(* Logix 5000 AddOnInstructionDefinition export Banner_IOLM_Param_A2_v4; software revision 36.00 *)

TYPE Banner_IOL_Port_v4 :   // UDT that has all of the data items necessary to communicate with a specific Port on a IO-Link Master
STRUCT
   Port_Controlled : INT;   // Each bit represents a port on an IO-Link Master. Set to 1 to tell AOI to control that port.
   Port_Activate : INT;   // Each bit represents a port on an IO-Link Master. When ON that port will process any commands in queue.
   Port_Read : INT;   // Each bit represents a port on an IO-Link Master. Used to determine when device AOI has requested a Read command.
   Port_Write : INT;   // Each bit represents a port on an IO-Link Master. Used to determine when device AOI has requested a Write command.
   Port_RW_Complete : INT;   // Each bit represents a port on an IO-Link Master. Tells device AOI that Read or Write request has been completed.
   Port_Device_Read : INT;
   Data_Transfer : SINT[190];   // Array to transfer data from IO-Master to device AOIs.
END_STRUCT
END_TYPE

TYPE Banner_IOLM_EL_v4 :   // Error Log for Messages to IOLM.
STRUCT
   RW : SINT;   // 0 = Read, 1 = Write.
   Port : SINT;   // Port number that generated error.
   Index : INT;   // IO-Link Index for generated error.
END_STRUCT
END_TYPE

TYPE Banner_IOLM_v4 :   // UDT to control IO-Link Masters.
STRUCT
   Message_Source_Data : SINT[190];
   Message_Destination_Data : SINT[190];
   Error_Log : Banner_IOLM_EL_v4[10];
   Error_Write_Retry : BOOL;
   Num_Error_MSGS : DINT;
   IO_Link_Master_Busy : BOOL;   // 0 = While waiting for a command, 1 = Processing command
   AOI_Reset : BOOL;
   Port_Data : Banner_IOL_Port_v4;   // All of the necessary data to work with the various ports of the IO-Link Master.
   Halt_Operation : BOOL;   // When parameter is 1 the AOI is halted as next available time frame.
   AOI_Halted : BOOL;   // AOI is in standby mode until Halt Operation tag is set back to 0.
END_STRUCT
END_TYPE

ADD_ON_INSTRUCTION Banner_IOLM_Param_A2_v4   (* revision 4.1, vendor Banner Engineering *)
// AOI that controls an Allen Bradley IO-Link Master with Banner devices for parameter data operations. Created for use with the 5032-8IOLM units only.
VAR_IN_OUT
   Message_Read : MESSAGE; {required}   // Message used to gather data from a device plugged into an Allen Bradley IO-Link Master.
   Message_Write : MESSAGE; {required}   // Message used to send parameter updates to a device plugged into an Allen Bradley IO-Link Master.
   IOLM : Banner_IOLM_v4; {required}
   ISDU_Path : STRING[8]; {required}
END_VAR
VAR_OUTPUT
   Done : BOOL; {visible}
   Busy : BOOL; {visible}
   Error : BOOL; {visible}
END_VAR
VAR
   Lock : DINT; {access None}
   Byte_Length : SINT; {access None}
   Current_Port : INT; {access None}   // Current port to communicate with via the IO-Link Master.
   Array_Index : DINT; {access None}
   Data_Index : DINT; {access None}
   Message_Timer : TIMER := (PRE := 100); {access None}
   Error_Index : DINT; {access None}
   Message_Timer2 : TIMER := (PRE := 5000); {access None}
   Temp_Index : INT; {access None}
END_VAR

ROUTINE Logic   (* ladder *)
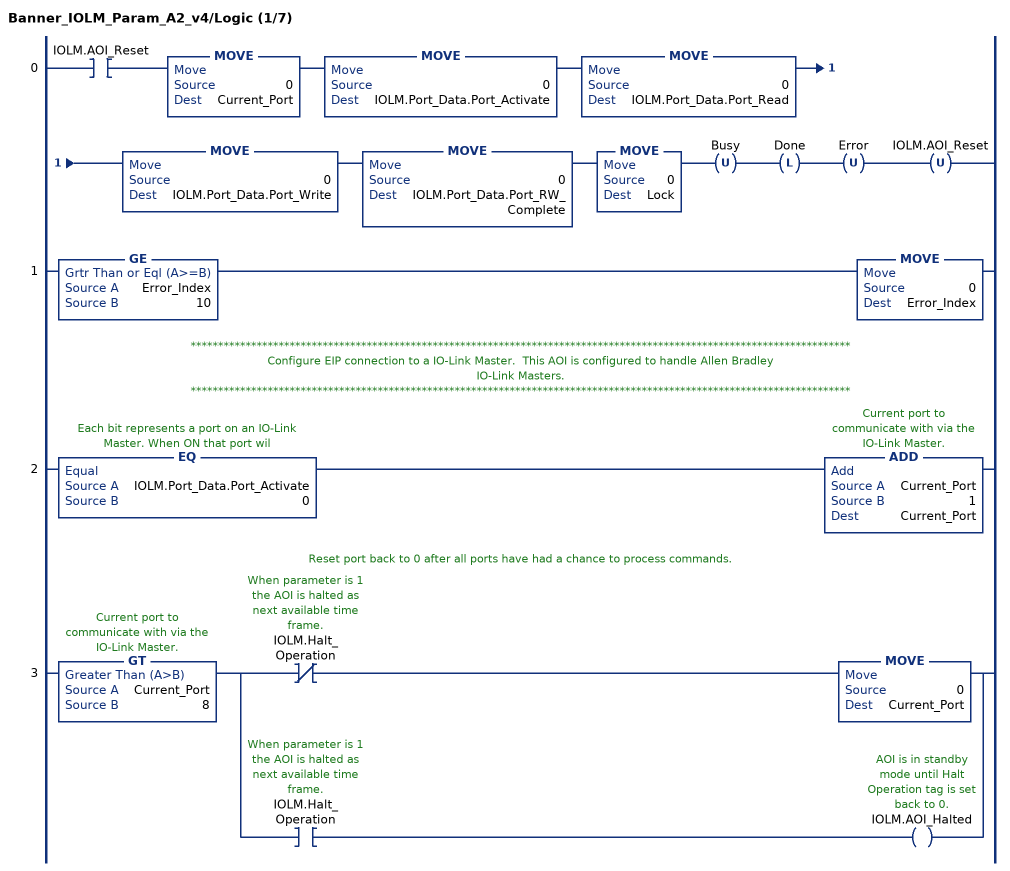
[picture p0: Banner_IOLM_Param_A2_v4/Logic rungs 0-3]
   0: XIC(IOLM.AOI_Reset)MOVE(0,Current_Port)MOVE(0,IOLM.Port_Data.Port_Activate)MOVE(0,IOLM.Port_Data.Port_Read)MOVE(0,IOLM.Port_Data.Port_Write)MOVE(0,IOLM.Port_Data.Port_RW_Complete)MOVE(0,Lock)OTU(Busy)OTL(Done)OTU(Error)OTU(IOLM.AOI_Reset);
   1: GE(Error_Index,10)MOVE(0,Error_Index);
   // ************************************************************************************************************************
   // Configure EIP connection to a IO-Link Master.  This AOI is configured to handle Allen Bradley
   // IO-Link Masters.
   // ************************************************************************************************************************
   2: EQ(IOLM.Port_Data.Port_Activate,0)ADD(Current_Port,1,Current_Port);
   // Reset port back to 0 after all ports have had a chance to process commands.
   3: GT(Current_Port,8)[XIO(IOLM.Halt_Operation) MOVE(0,Current_Port) ,XIC(IOLM.Halt_Operation) OTE(IOLM.AOI_Halted) ];
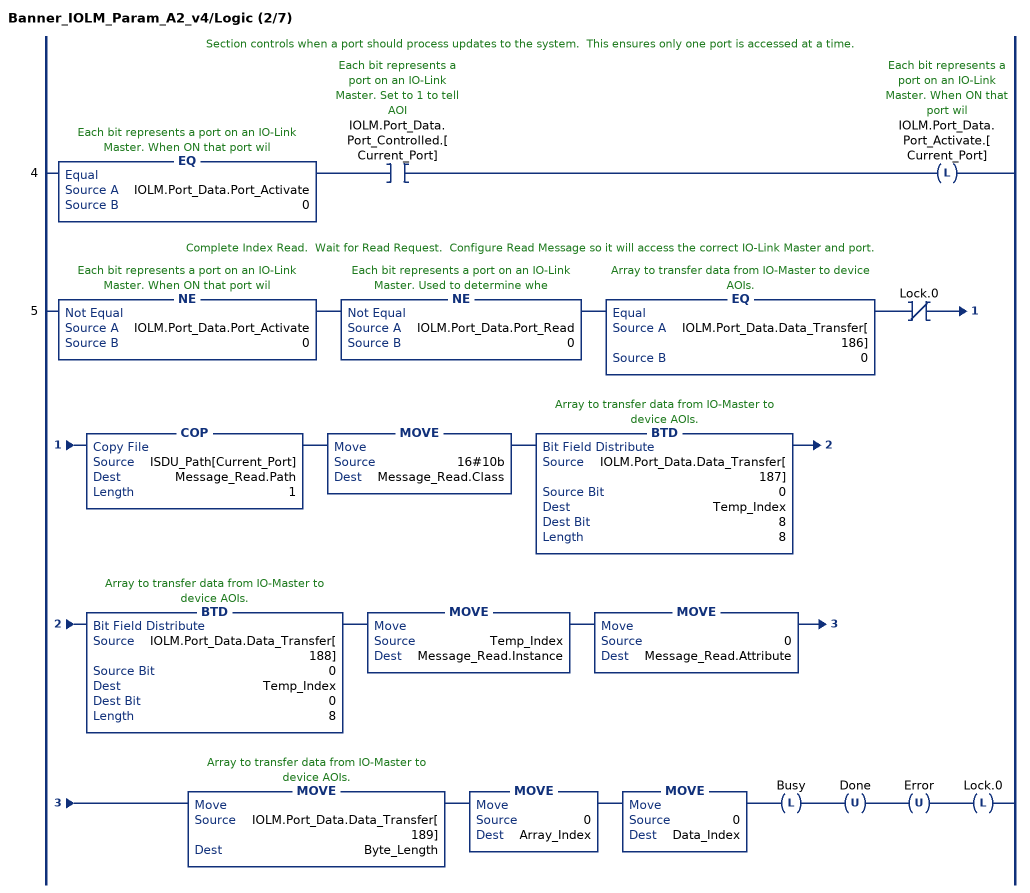
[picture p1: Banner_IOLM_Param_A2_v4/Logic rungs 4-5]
   // Section controls when a port should process updates to the system.  This ensures only one port is accessed at a time.
   4: EQ(IOLM.Port_Data.Port_Activate,0)XIC(IOLM.Port_Data.Port_Controlled.[Current_Port])OTL(IOLM.Port_Data.Port_Activate.[Current_Port]);
   // Complete Index Read.  Wait for Read Request.  Configure Read Message so it will access the correct IO-Link Master and port.
   5: NE(IOLM.Port_Data.Port_Activate,0)NE(IOLM.Port_Data.Port_Read,0)EQ(IOLM.Port_Data.Data_Transfer[186],0)XIO(Lock.0)COP(ISDU_Path[Current_Port],Message_Read.Path,1)MOVE(16#10b,Message_Read.Class)BTD(IOLM.Port_Data.Data_Transfer[187],0,Temp_Index,8,8)BTD(IOLM.Port_Data.Data_Transfer[188],0,Temp_Index,0,8)MOVE(Temp_Index,Message_Read.Instance)MOVE(0,Message_Read.Attribute)MOVE(IOLM.Port_Data.Data_Transfer[189],Byte_Length)MOVE(0,Array_Index)MOVE(0,Data_Index)OTL(Busy)OTU(Done)OTU(Error)OTL(Lock.0);
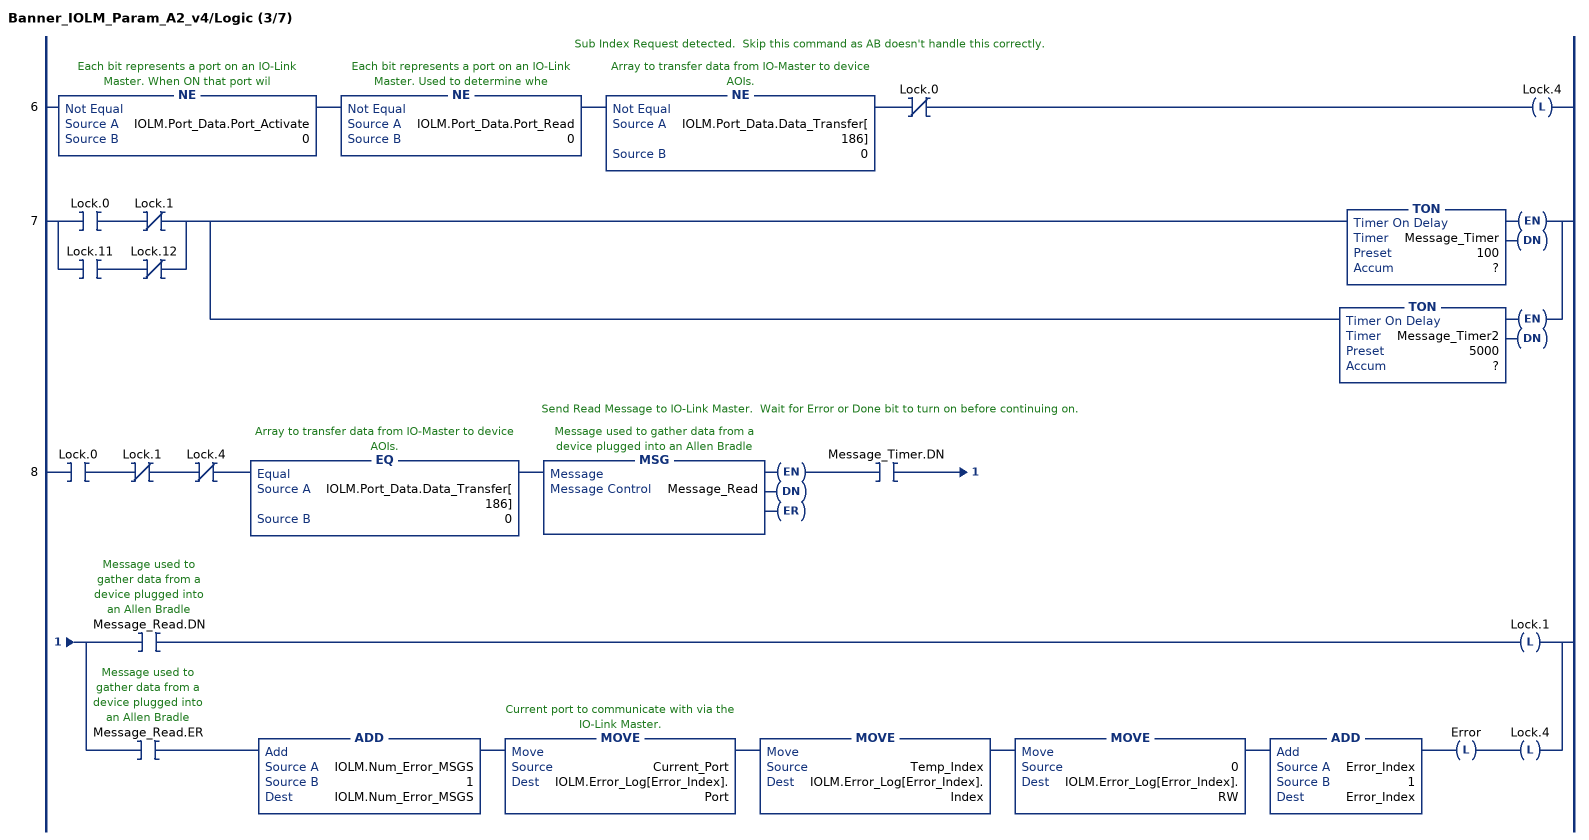
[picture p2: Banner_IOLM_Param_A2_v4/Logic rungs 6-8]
   // Sub Index Request detected.  Skip this command as AB doesn't handle this correctly.
   6: NE(IOLM.Port_Data.Port_Activate,0)NE(IOLM.Port_Data.Port_Read,0)NE(IOLM.Port_Data.Data_Transfer[186],0)XIO(Lock.0)OTL(Lock.4);
   7: [XIC(Lock.0) XIO(Lock.1) ,XIC(Lock.11) XIO(Lock.12) ][TON(Message_Timer,?,?) ,TON(Message_Timer2,?,?) ];
   // Send Read Message to IO-Link Master.  Wait for Error or Done bit to turn on before continuing on.
   8: XIC(Lock.0)XIO(Lock.1)XIO(Lock.4)EQ(IOLM.Port_Data.Data_Transfer[186],0)MSG(Message_Read)XIC(Message_Timer.DN)[XIC(Message_Read.DN) OTL(Lock.1) ,XIC(Message_Read.ER) ADD(IOLM.Num_Error_MSGS,1,IOLM.Num_Error_MSGS) MOVE(Current_Port,IOLM.Error_Log[Error_Index].Port) MOVE(Temp_Index,IOLM.Error_Log[Error_Index].Index) MOVE(0,IOLM.Error_Log[Error_Index].RW) ADD(Error_Index,1,Error_Index) OTL(Error) OTL(Lock.4) ];
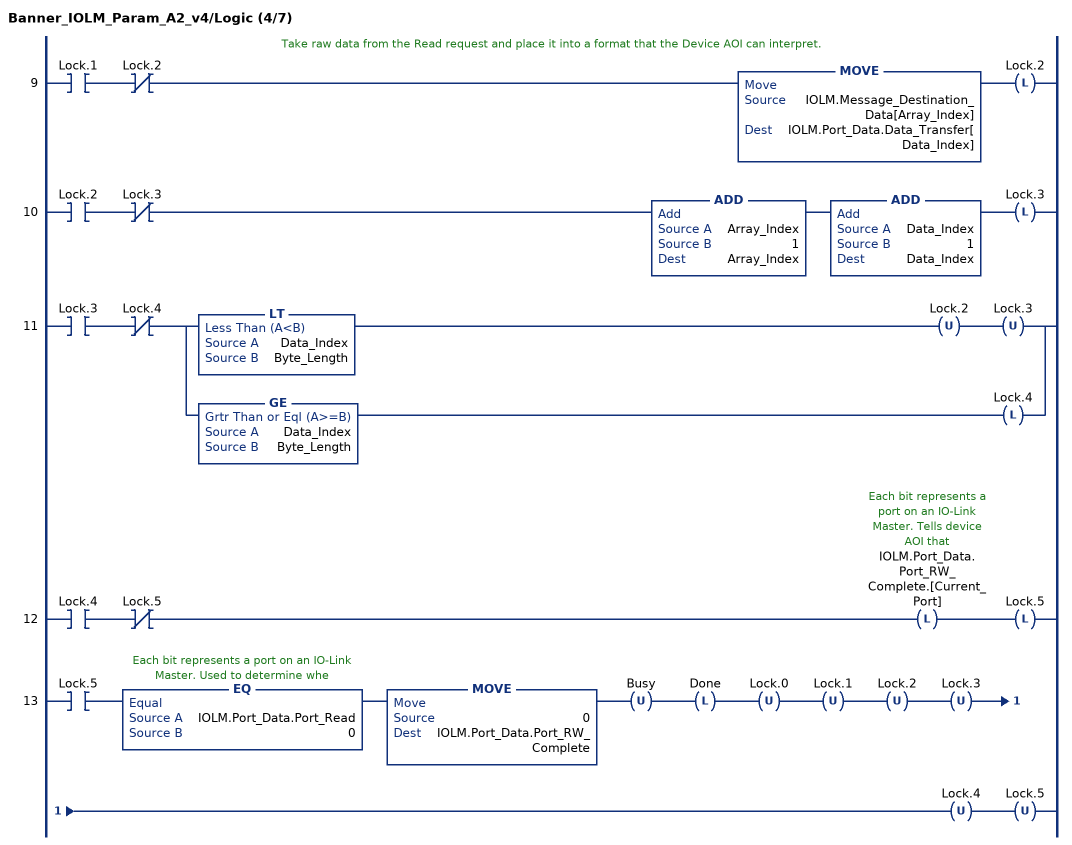
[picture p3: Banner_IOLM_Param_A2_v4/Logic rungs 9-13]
   // Take raw data from the Read request and place it into a format that the Device AOI can interpret.
   9: XIC(Lock.1)XIO(Lock.2)MOVE(IOLM.Message_Destination_Data[Array_Index],IOLM.Port_Data.Data_Transfer[Data_Index])OTL(Lock.2);
   10: XIC(Lock.2)XIO(Lock.3)ADD(Array_Index,1,Array_Index)ADD(Data_Index,1,Data_Index)OTL(Lock.3);
   11: XIC(Lock.3)XIO(Lock.4)[LT(Data_Index,Byte_Length) OTU(Lock.2) OTU(Lock.3) ,GE(Data_Index,Byte_Length) OTL(Lock.4) ];
   12: XIC(Lock.4)XIO(Lock.5)OTL(IOLM.Port_Data.Port_RW_Complete.[Current_Port])OTL(Lock.5);
   13: XIC(Lock.5)EQ(IOLM.Port_Data.Port_Read,0)MOVE(0,IOLM.Port_Data.Port_RW_Complete)OTU(Busy)OTL(Done)OTU(Lock.0)OTU(Lock.1)OTU(Lock.2)OTU(Lock.3)OTU(Lock.4)OTU(Lock.5);
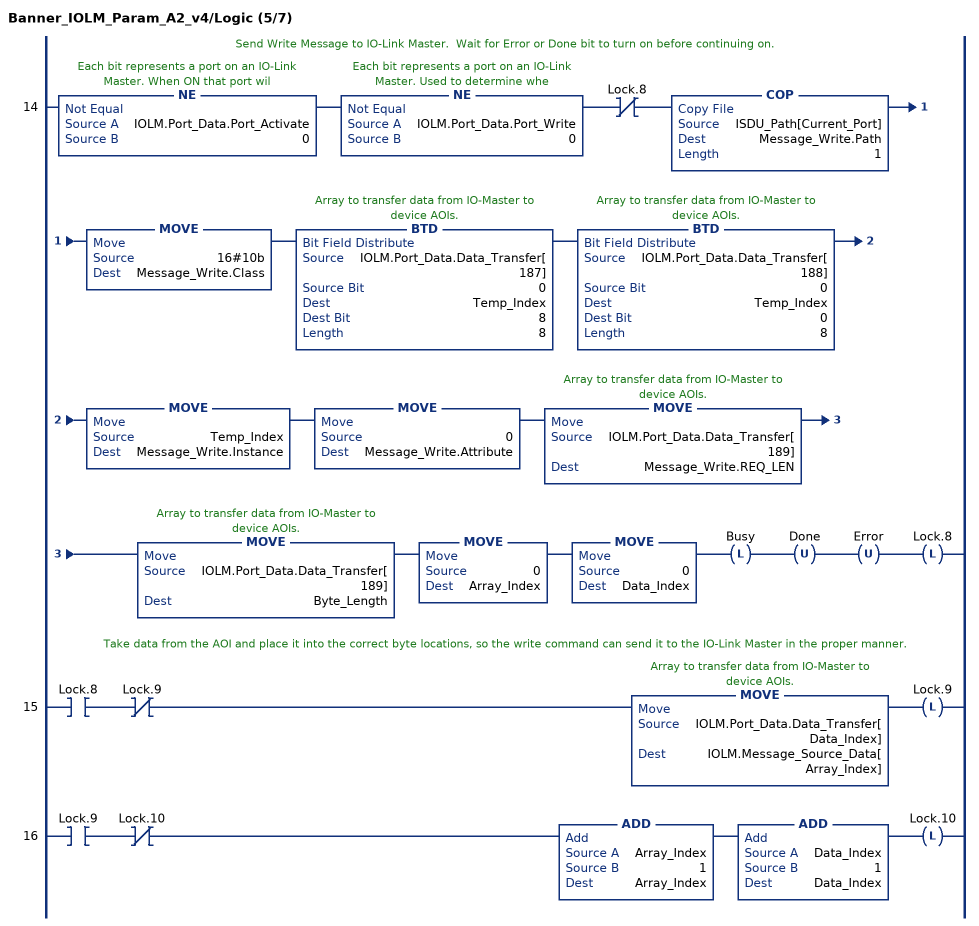
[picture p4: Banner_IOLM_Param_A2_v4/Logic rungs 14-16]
   // Send Write Message to IO-Link Master.  Wait for Error or Done bit to turn on before continuing on.
   14: NE(IOLM.Port_Data.Port_Activate,0)NE(IOLM.Port_Data.Port_Write,0)XIO(Lock.8)COP(ISDU_Path[Current_Port],Message_Write.Path,1)MOVE(16#10b,Message_Write.Class)BTD(IOLM.Port_Data.Data_Transfer[187],0,Temp_Index,8,8)BTD(IOLM.Port_Data.Data_Transfer[188],0,Temp_Index,0,8)MOVE(Temp_Index,Message_Write.Instance)MOVE(0,Message_Write.Attribute)MOVE(IOLM.Port_Data.Data_Transfer[189],Message_Write.REQ_LEN)MOVE(IOLM.Port_Data.Data_Transfer[189],Byte_Length)MOVE(0,Array_Index)MOVE(0,Data_Index)OTL(Busy)OTU(Done)OTU(Error)OTL(Lock.8);
   // Take data from the AOI and place it into the correct byte locations, so the write command can send it to the IO-Link Master in the proper manner.
   15: XIC(Lock.8)XIO(Lock.9)MOVE(IOLM.Port_Data.Data_Transfer[Data_Index],IOLM.Message_Source_Data[Array_Index])OTL(Lock.9);
   16: XIC(Lock.9)XIO(Lock.10)ADD(Array_Index,1,Array_Index)ADD(Data_Index,1,Data_Index)OTL(Lock.10);
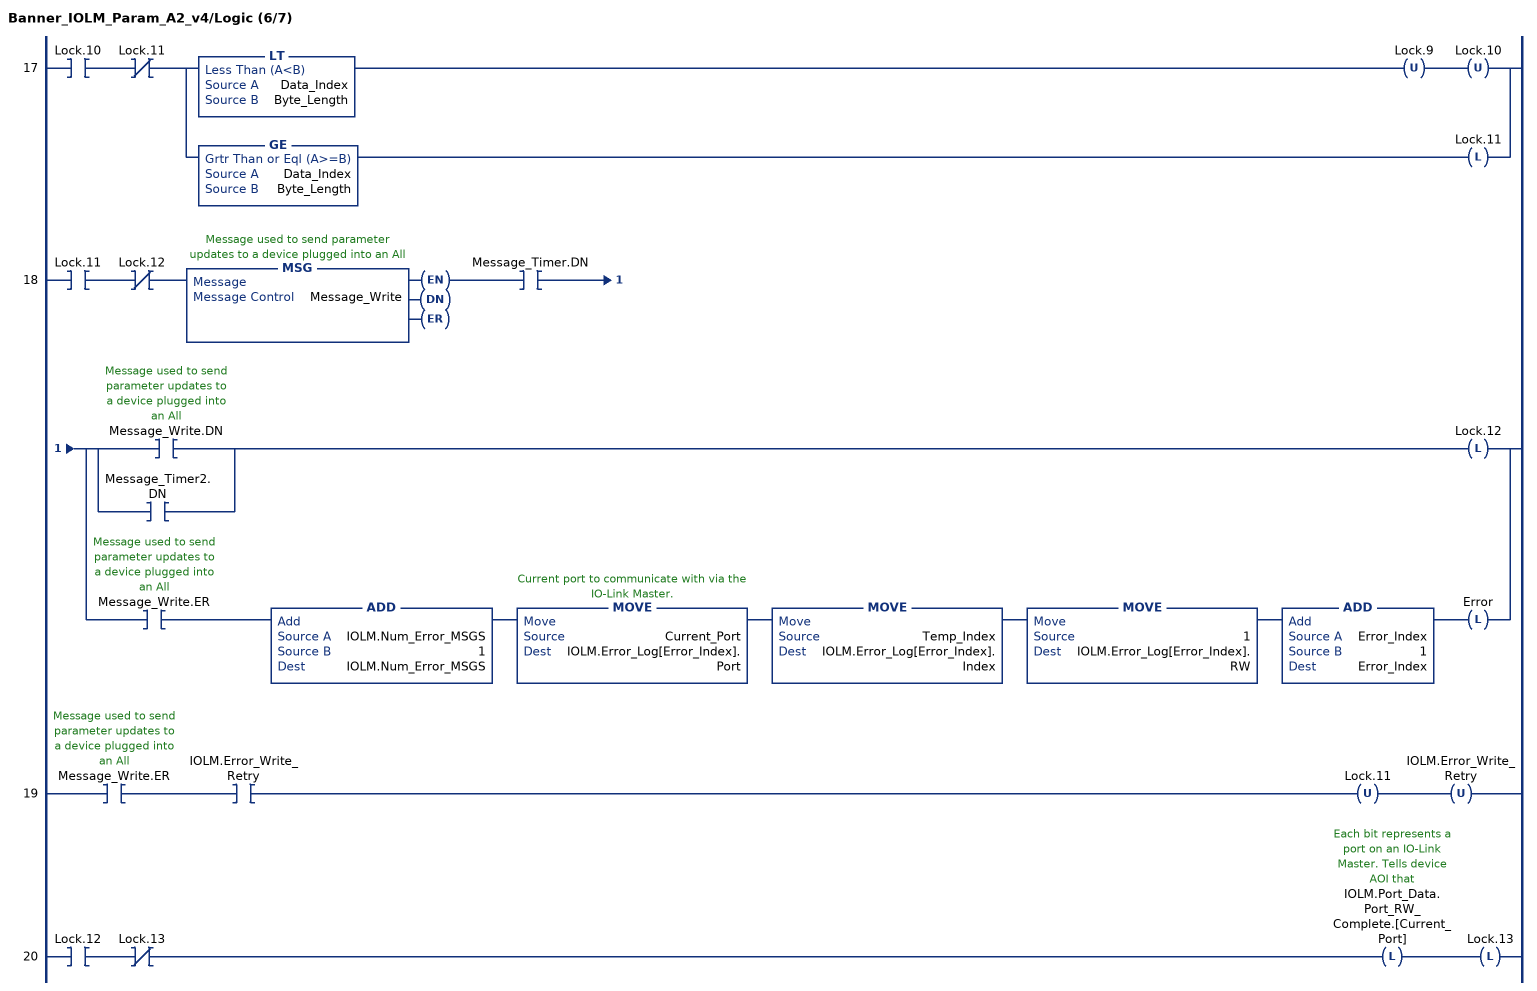
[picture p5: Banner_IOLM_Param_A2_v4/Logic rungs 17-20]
   17: XIC(Lock.10)XIO(Lock.11)[LT(Data_Index,Byte_Length) OTU(Lock.9) OTU(Lock.10) ,GE(Data_Index,Byte_Length) OTL(Lock.11) ];
   18: XIC(Lock.11)XIO(Lock.12)MSG(Message_Write)XIC(Message_Timer.DN)[[XIC(Message_Write.DN) ,XIC(Message_Timer2.DN) ] OTL(Lock.12) ,XIC(Message_Write.ER) ADD(IOLM.Num_Error_MSGS,1,IOLM.Num_Error_MSGS) MOVE(Current_Port,IOLM.Error_Log[Error_Index].Port) MOVE(Temp_Index,IOLM.Error_Log[Error_Index].Index) MOVE(1,IOLM.Error_Log[Error_Index].RW) ADD(Error_Index,1,Error_Index) OTL(Error) ];
   19: XIC(Message_Write.ER)XIC(IOLM.Error_Write_Retry)OTU(Lock.11)OTU(IOLM.Error_Write_Retry);
   20: XIC(Lock.12)XIO(Lock.13)OTL(IOLM.Port_Data.Port_RW_Complete.[Current_Port])OTL(Lock.13);
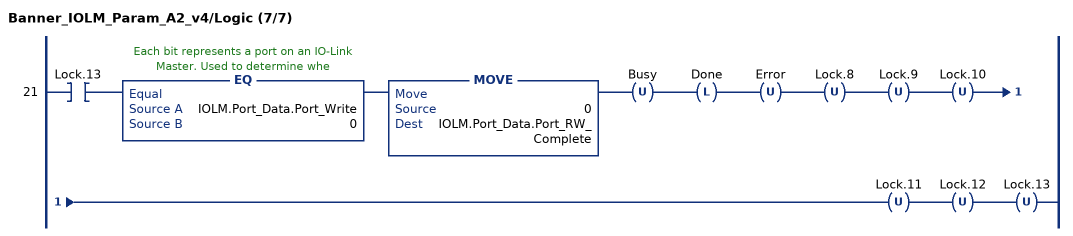
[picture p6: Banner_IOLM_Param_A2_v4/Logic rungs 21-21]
   21: XIC(Lock.13)EQ(IOLM.Port_Data.Port_Write,0)MOVE(0,IOLM.Port_Data.Port_RW_Complete)OTU(Busy)OTL(Done)OTU(Error)OTU(Lock.8)OTU(Lock.9)OTU(Lock.10)OTU(Lock.11)OTU(Lock.12)OTU(Lock.13);
END_ROUTINE
END_ADD_ON_INSTRUCTION
